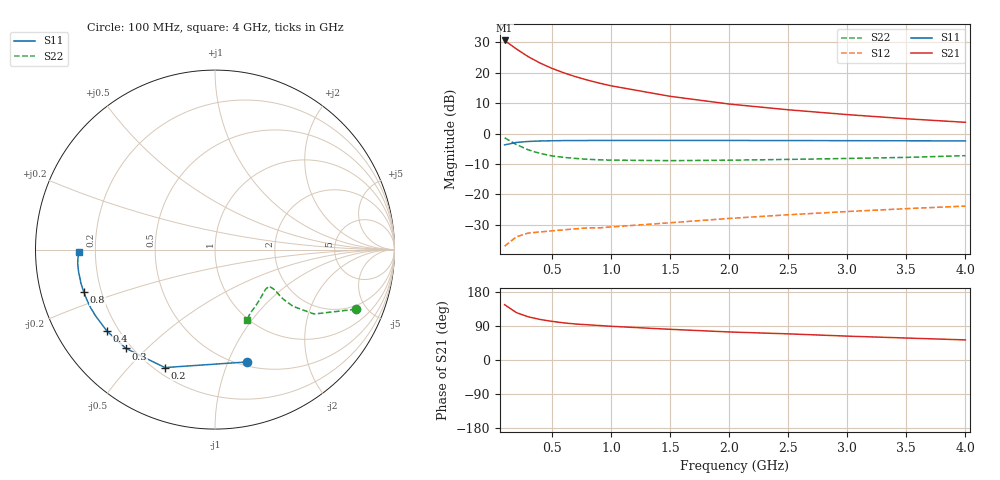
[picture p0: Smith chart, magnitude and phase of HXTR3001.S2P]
! HXTR-3001 Common Emitter
! Vce=15v Ic=15mA
# ghz s ma r 50
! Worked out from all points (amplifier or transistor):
!   16 points, 100 MHz to 4 GHz, reference 50 ohm
!   highest |S21| = 30.6 dB at 100 MHz (marker M1)
!   |S21| within 3 dB of that: start of sweep to 207.9 MHz
!   unconditionally stable (mu >= 1): 1.306 GHz to end of sweep
!   at 300 MHz: K = 0.29, MSG = 29.0 dB, |S12| = -32.8 dB
!   at 900 MHz: K = 0.80, MSG = 23.8 dB, |S12| = -31.1 dB
!   at 4 GHz: K = 1.51, MAG = 9.6 dB, |S12| = -23.9 dB
!   S11 on the Smith chart (normalised r, x): 100 MHz: 0.54, -1.18; 200 MHz: 0.24, -0.64; 300 MHz: 0.18, -0.43; 400 MHz: 0.16, -0.33; 800 MHz: 0.13, -0.16; 4 GHz: 0.14, -0.01
0.1  0.651 -74.0  34.04 146.0  0.014 59.0  0.851 -23.0
0.2  0.714 -113.0  24.66 125.0  0.02 43.0  0.659 -33.0
0.3  0.741 -132.0  18.41 114.0  0.023 36.0  0.539 -36.0
0.4  0.754 -143.0  14.46 107.0  0.024 33.0  0.471 -36.0
0.5  0.761 -151.0  11.84 102.0  0.025 31.0  0.429 -35.0
0.6  0.765 -155.0  10 98.0  0.026 32.0  0.405 -34.0
0.7  0.767 -159.0  8.63 95.0  0.027 32.0  0.389 -34.0
0.8  0.768 -162.0  7.59 93.0  0.028 33.0  0.377 -34.0
0.9  0.769 -164.0  6.77 91.0  0.028 34.0  0.37 -34.0
1  0.77 -166.0  6.11 89.0  0.029 35.0  0.365 -34.0
1.5  0.77 -171.0  4.1 81.0  0.034 41.0  0.358 -38.0
2  0.769 -174.0  3.06 74.0  0.04 44.0  0.364 -43.0
2.5  0.766 -176.0  2.46 69.0  0.046 47.0  0.375 -49.0
3  0.763 -177.0  2.05 63.0  0.052 48.0  0.389 -55.0
3.5  0.76 -178.0  1.75 58.0  0.058 48.0  0.405 -61.0
4  0.756 -179.0  1.53 53.0  0.064 48.0  0.432 -66.0
